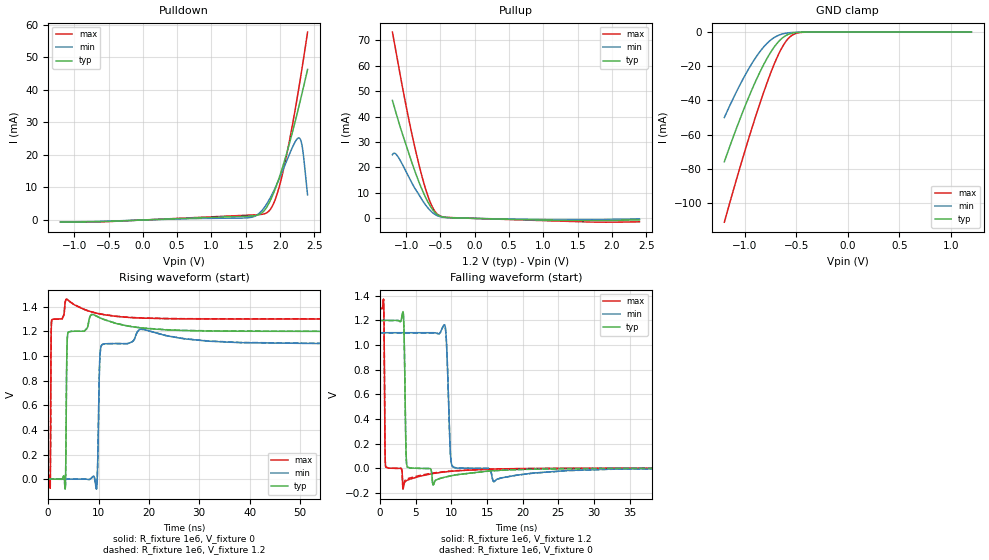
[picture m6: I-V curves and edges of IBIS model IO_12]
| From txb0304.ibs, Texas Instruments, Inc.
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[Model]   IO_12
Model_type  3-state
Enable   Active-High
Vref =   0
Rref =   1e6
Cref =   100p
Vmeas =   0.6
| variable   typ   min   max
C_comp   3.93pF   3.64pF   4.13pF
| C_pullup   4.20pF   3.84pF   4.44pF
| C_pulldown   4.19pF   3.83pF   4.36pF
| C_tri-state   3.93pF   3.64pF   4.13pF
[Temperature Range]   40   100   -40
| Ambient temperature   25   85   -40
[Voltage range]   1.2   1.1   1.3
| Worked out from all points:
|   slope of the pulldown table from 0 to 0.18 V, typ, clamps not added: 1.19 kohm
|   slope of the pullup table from 0 to 0.18 V, typ, clamps not added: 1.38 kohm
|   GND clamp passes 1 mA (typ) near -0.56 V on its own axis
|   rising waveform, R_fixture 1e6, V_fixture 0: 20-80 % time 166ps typ, 297ps min, 95.8ps max; typ from 0 V to 1.2 V
|   falling waveform, R_fixture 1e6, V_fixture 1.2: 20-80 % time 189ps typ, 372ps min, 99.7ps max; typ from 1.2 V to 0.001 V
|   rising waveform, R_fixture 1e6, V_fixture 1.2: 20-80 % time 167ps typ, 298ps min, 95.9ps max; typ from 0.001 V to 1.2 V
|   falling waveform, R_fixture 1e6, V_fixture 0: 20-80 % time 189ps typ, 372ps min, 99.7ps max; typ from 1.2 V to 0 V
[GND Clamp]
| IO_12
|   Voltage   I(typ)   I(min)   I(max)
-1.2V     -75.93mA   -50.03mA   -111.3mA
-1.09V    -57.58mA   -35.88mA   -87.94mA
-990mV    -42.07mA   -24.33mA   -67.55mA
-900mV    -29.33mA   -15.35mA   -50.15mA
-820mV    -19.29mA   -8.867mA   -35.65mA
-740mV    -10.89mA   -4.215mA   -22.43mA
-670mV    -5.38mA    -1.799mA   -12.58mA
-610mV    -2.329mA   -749.6uA   -6.159mA
-555mV    -857.1uA   -301.9uA   -2.435mA
-495mV    -231uA     -94.89uA   -625.1uA
-400mV    -20.35uA   -9.848uA   -38.49uA
1.2V      331.2pA    18.1nA     22.5pA
[Pulldown]
| IO_12
|   Voltage   I(typ)   I(min)   I(max)
-1.2V     -625uA     -574.3uA   -672.8uA
1.535V    1.18mA     686.1uA    1.486mA
1.71V     1.854mA    2.348mA    1.687mA
1.82V     4.479mA    5.466mA    2.445mA
1.915V    8.825mA    9.289mA    5.571mA
2.01V     14.5mA     13.79mA    12.03mA
2.13V     23.08mA    19.92mA    23.71mA
2.22V     30.33mA    24.06mA    34mA
2.27V     34.6mA     25.23mA    40.2mA
2.3V      37.23mA    24.55mA    44.08mA
2.325V    39.45mA    22.18mA    47.39mA
2.4V      46.28mA    7.742mA    57.77mA
[Pullup]
| IO_12
|   Voltage   I(typ)   I(min)   I(max)
-1.2V     46.31mA    25mA       73.14mA
-1.165V   43.04mA    25.53mA    67.97mA
-1.12V    38.89mA    24.24mA    61.23mA
-955mV    25.03mA    15.94mA    38.06mA
-805mV    13.72mA    8.923mA    20.22mA
-730mV    9.015mA    5.778mA    12.71mA
-660mV    5.366mA    3.412mA    7.076mA
-595mV    2.811mA    1.841mA    3.383mA
-535mV    1.347mA    952.8uA    1.454mA
-395mV    343.4uA    288.9uA    381.7uA
650mV     -458.8uA   -339.1uA   -572.7uA
2.4V      -573.8uA   -201.8uA   -1.327mA
[Ramp]
| IO_12
| variable   typ   min   max
dV/dt_r   0.85/2.23E-10   0.78/3.82E-10   0.92/1.45E-10
dV/dt_f   0.84/2.50E-10   0.76/4.49E-10   0.92/1.32E-10
R_load = 1e6
[Rising Waveform]
| IO_12
R_fixture =   1e6
C_fixture =   0
L_fixture =   0
V_fixture =   0
V_fixture_min = 0
V_fixture_max = 0
|   Time   V(typ)   V(min)   V(max)
0s        353.9nV    2.094uV    36.67nV
413ps     298.3nV    2.094uV    -74.24mV
581ps     231.1nV    2.094uV    1.125V
677ps     200.9nV    2.094uV    1.282V
3.389ns   -74.86mV   2.031uV    1.433V
3.653ns   839.8mV    2.008uV    1.459V
9.605ns   1.322V     -80.22mV   1.346V
10.49ns   1.305V     1.074V     1.338V
18.32ns   1.227V     1.215V     1.306V
115.8ns   1.198V     1.098V     1.299V
[Falling Waveform]
| IO_12
R_fixture =   1e6
C_fixture =   0
L_fixture =   0
V_fixture =   1.2
V_fixture_min = 1.1
V_fixture_max = 1.3
|   Time   V(typ)   V(min)   V(max)
0s        1.2V       1.1V       1.3V
509ps     1.2V       1.1V       1.34V
773ps     1.2V       1.1V       16.3mV
3.221ns   1.271V     1.1V       -168.5mV
3.725ns   34.9mV     1.1V       -98.4mV
7.421ns   -135mV     1.1V       -42.06mV
9.149ns   -70.33mV   1.145V     -28.33mV
10.09ns   -58.59mV   23.77mV    -22.81mV
15.97ns   -18.17mV   -107.8mV   -5.306mV
115.8ns   1.421mV    1.619mV    1.312mV
[Rising Waveform]
| IO_12
R_fixture =   1e6
C_fixture =   0
L_fixture =   0
V_fixture =   1.2
V_fixture_min = 1.1
V_fixture_max = 1.3
|   Time   V(typ)   V(min)   V(max)
0s        1.421mV    1.618mV    1.31mV
413ps     1.421mV    1.618mV    -72.93mV
581ps     1.421mV    1.618mV    1.125V
677ps     1.421mV    1.618mV    1.282V
3.389ns   -73.36mV   1.618mV    1.435V
3.653ns   840.9mV    1.618mV    1.46V
9.605ns   1.322V     -78.33mV   1.347V
10.49ns   1.305V     1.074V     1.339V
18.32ns   1.228V     1.216V     1.308V
115.8ns   1.2V       1.1V       1.3V
[Falling Waveform]
| IO_12
R_fixture =   1e6
C_fixture =   0
L_fixture =   0
V_fixture =   0
V_fixture_min = 0
V_fixture_max = 0
|   Time   V(typ)   V(min)   V(max)
0s        1.198V     1.098V     1.299V
509ps     1.198V     1.098V     1.338V
773ps     1.198V     1.098V     16.25mV
3.221ns   1.269V     1.098V     -159.4mV
3.725ns   34.71mV    1.098V     -87.39mV
7.421ns   -135.1mV   1.098V     -37.98mV
9.149ns   -70.76mV   1.143V     -25.95mV
10.09ns   -59.18mV   23.65mV    -21.12mV
15.97ns   -19.31mV   -107.9mV   -5.789mV
115.8ns   233.7nV    4.173uV    1.287uV
